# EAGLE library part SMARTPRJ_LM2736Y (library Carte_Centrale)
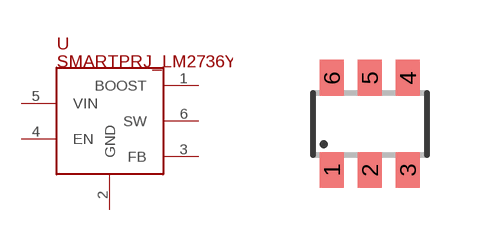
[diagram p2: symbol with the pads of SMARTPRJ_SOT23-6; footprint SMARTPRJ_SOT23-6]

Designator prefix -

## SMARTPRJ_LM2736Y  [SMARTPRJ_SOT23-6]
1  BOOST  in
2  GND  pwr
3  FB  in
4  EN  in
5  VIN  in
6  SW  out

## Footprint SMARTPRJ_SOT23-6 (pad centres in mm)
Small Outline Transistor 6 lead
smd 0.6 x 0.9: 1 -0.95,-1.15; 2 0,-1.15; 3 0.95,-1.15; 4 0.95,1.15; 5 0,1.15; 6 -0.95,1.15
